PROGRAM MAIN
VAR
	fbMBUS_REL_PadIn4	:	FB_MBUS_REL_PadIn4;
	usiAddress			:	USINT;
	bDataIn1			: 	BOOL;
	bDataIn2			:	BOOL;
	bDataIn3			:	BOOL;
	bDataIn4			:	BOOL;
END_VAR

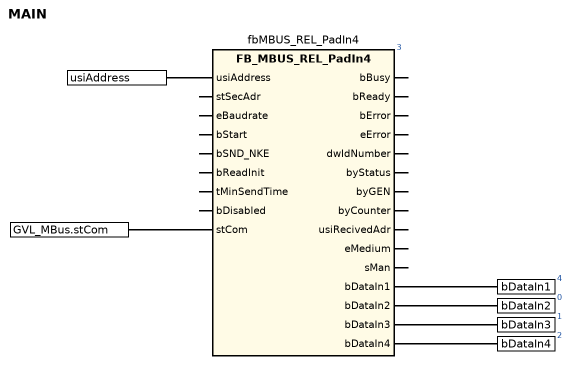
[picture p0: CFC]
bDataIn2 := fbMBUS_REL_PadIn4.bDataIn2;
bDataIn3 := fbMBUS_REL_PadIn4.bDataIn3;
bDataIn4 := fbMBUS_REL_PadIn4.bDataIn4;
fbMBUS_REL_PadIn4(usiAddress := usiAddress, stCom := GVL_MBus.stCom); // FB_MBUS_REL_PadIn4
bDataIn1 := fbMBUS_REL_PadIn4.bDataIn1;

END_PROGRAM
